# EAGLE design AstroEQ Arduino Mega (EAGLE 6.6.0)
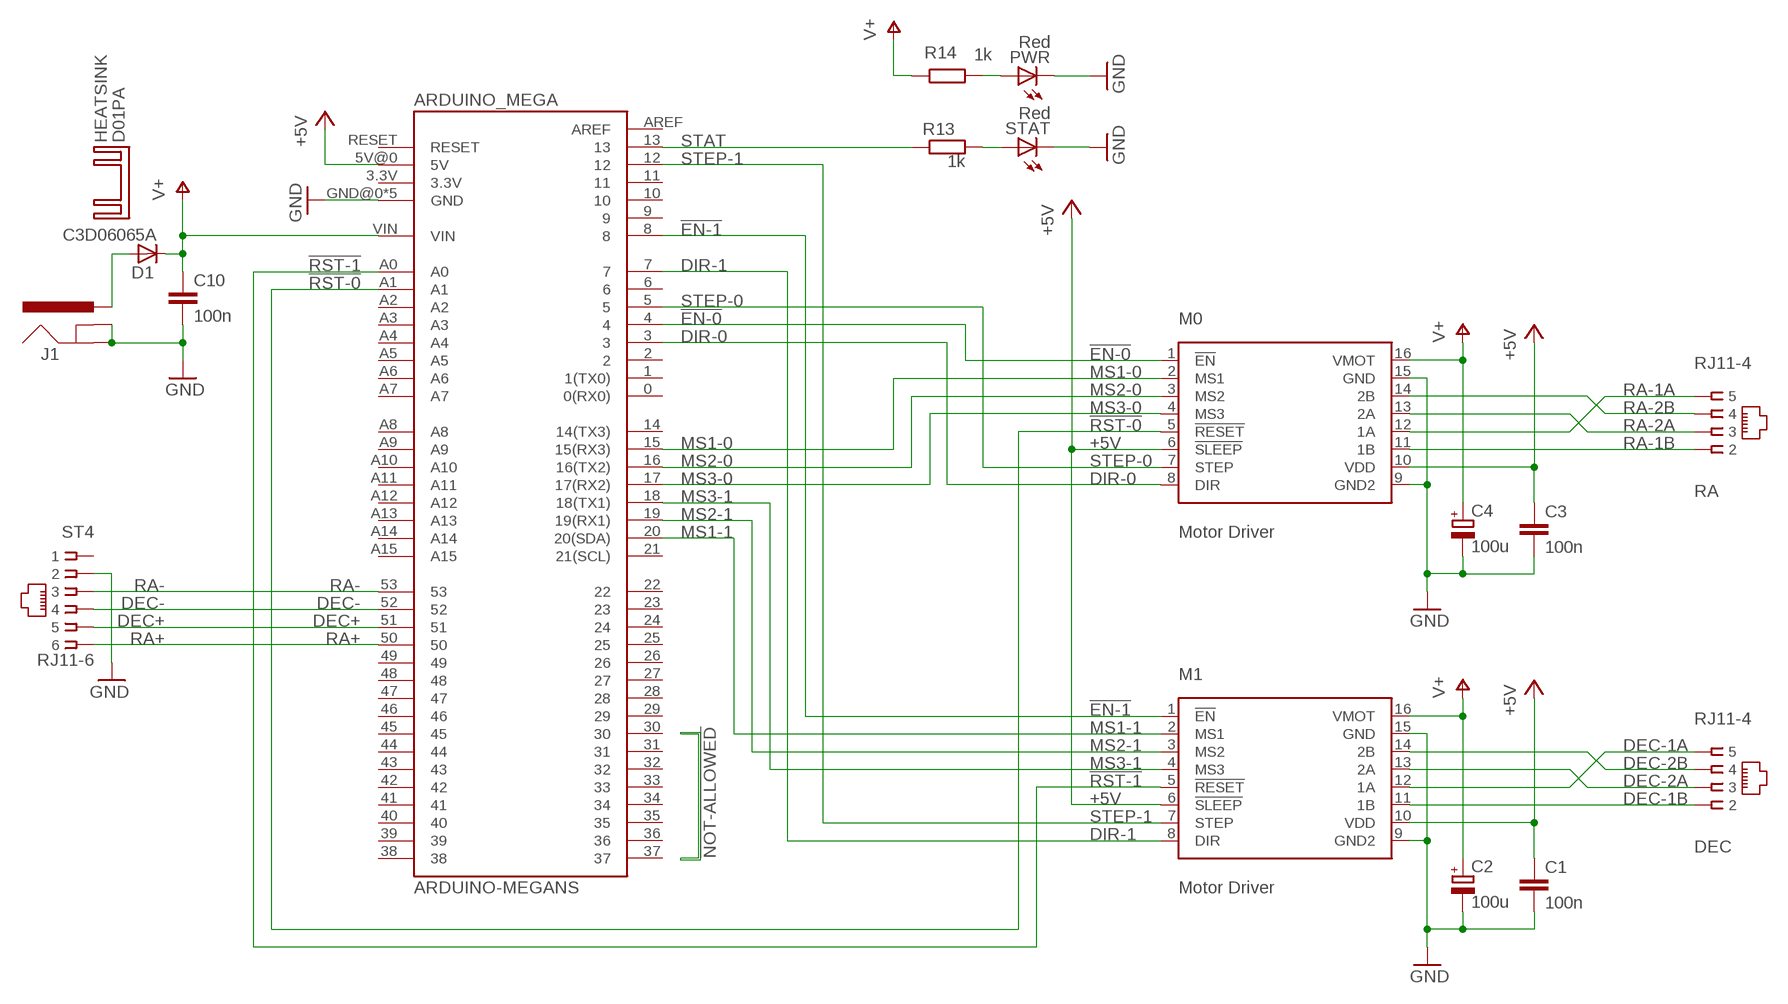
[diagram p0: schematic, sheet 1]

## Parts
ARDUINO_MEGA  ARDUINO-MEGANS  [ARDUINO_MEGA_NS]
C1  100n  C-EU025-024X044  [C025-024X044]
C2  100u  CPOL-EUE2.5-7  [E2,5-7]
C3  100n  C-EU025-024X044  [C025-024X044]
C4  100u  CPOL-EUE2.5-7  [E2,5-7]
C10  100n  C-EU025-024X044  [C025-024X044]
D1  C3D06065A  MUR820VERT  [TO220ACS]
DEC  RJ11-4  [RJ11-NO_SHIELD-4]
HEATSINK  D01PA  [D01PA]
J1  POWER_JACKPTH  [POWER_JACK_PTH]
M0  Motor Driver  A4983CARRIER  [DIP16-W]
M1  Motor Driver  A4983CARRIER  [DIP16-W]
PWR  Red  LED3MM  [LED3MM]
R13  1k  R-EU_0204/5  [0204/5]
R14  1k  R-EU_0204/7  [0204/7]
RA  RJ11-4  [RJ11-NO_SHIELD-4]
ST4  RJ11-6  RJ11-2L-B  [RJ11-NO_SHIELD]
STAT  Red  LED3MM  [LED3MM]

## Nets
!EN-0: ARDUINO_MEGA.4 M0.1(!EN)
!EN-1: ARDUINO_MEGA.8 M1.1(!EN)
!RST-0: ARDUINO_MEGA.A1 M0.5(!RESET)
!RST-1: ARDUINO_MEGA.A0 M1.5(!RESET)
+5V: ARDUINO_MEGA.5V@0(5V) C1.1 C3.1 M0.6(!SLEEP) M0.10(VDD) M1.6(!SLEEP) M1.10(VDD)
DEC+: ARDUINO_MEGA.51 ST4.5
DEC-: ARDUINO_MEGA.52 ST4.4
DEC-1A: DEC.5 M1.12(1A)
DEC-1B: DEC.2 M1.11(1B)
DEC-2A: DEC.3 M1.13(2A)
DEC-2B: DEC.4 M1.14(2B)
DIR-0: ARDUINO_MEGA.3 M0.8(DIR)
DIR-1: ARDUINO_MEGA.7 M1.8(DIR)
GND: ARDUINO_MEGA.GND@0(GND) ARDUINO_MEGA.GND@1(GND) ARDUINO_MEGA.GND@2(GND) ARDUINO_MEGA.GND@3(GND) ARDUINO_MEGA.GND@4(GND) C1.2 C2.- C3.2 C4.- C10.2 J1.GND J1.GNDBREAK M0.9(GND2) M0.15(GND) M1.9(GND2) M1.15(GND) PWR.K(C) ST4.2 STAT.K(C)
MS1-0: ARDUINO_MEGA.15(15(RX3)) M0.2(MS1)
MS1-1: ARDUINO_MEGA.20(20(SDA)) M1.2(MS1)
MS2-0: ARDUINO_MEGA.16(16(TX2)) M0.3(MS2)
MS2-1: ARDUINO_MEGA.19(19(RX1)) M1.3(MS2)
MS3-0: ARDUINO_MEGA.17(17(RX2)) M0.4(MS3)
MS3-1: ARDUINO_MEGA.18(18(TX1)) M1.4(MS3)
PWRLED: PWR.A R14.2
RA+: ARDUINO_MEGA.50 ST4.6
RA-: ARDUINO_MEGA.53 ST4.3
RA-1A: M0.12(1A) RA.5
RA-1B: M0.11(1B) RA.2
RA-2A: M0.13(2A) RA.3
RA-2B: M0.14(2B) RA.4
STAT: ARDUINO_MEGA.13 R13.1
STATLED: R13.2 STAT.A
STEP-0: ARDUINO_MEGA.5 M0.7(STEP)
STEP-1: ARDUINO_MEGA.12 M1.7(STEP)
V+: ARDUINO_MEGA.VIN C2.+ C4.+ C10.1 D1.C M0.16(VMOT) M1.16(VMOT) R14.1
VIN: D1.A J1.PWR
Unconnected: ARDUINO_MEGA.0(0(RX0)) ARDUINO_MEGA.1(1(TX0)) ARDUINO_MEGA.2 ARDUINO_MEGA.3.3V ARDUINO_MEGA.6 ARDUINO_MEGA.9 ARDUINO_MEGA.10 ARDUINO_MEGA.11 ARDUINO_MEGA.14(14(TX3)) ARDUINO_MEGA.21(21(SCL)) ARDUINO_MEGA.22 ARDUINO_MEGA.23 ARDUINO_MEGA.24 ARDUINO_MEGA.25 ARDUINO_MEGA.26 ARDUINO_MEGA.27 ARDUINO_MEGA.28 ARDUINO_MEGA.29 ARDUINO_MEGA.30 ARDUINO_MEGA.31 ARDUINO_MEGA.32 ARDUINO_MEGA.33 ARDUINO_MEGA.34 ARDUINO_MEGA.35 ARDUINO_MEGA.36 ARDUINO_MEGA.37 ARDUINO_MEGA.38 ARDUINO_MEGA.39 ARDUINO_MEGA.40 ARDUINO_MEGA.41 ARDUINO_MEGA.42 ARDUINO_MEGA.43 ARDUINO_MEGA.44 ARDUINO_MEGA.45 ARDUINO_MEGA.46 ARDUINO_MEGA.47 ARDUINO_MEGA.48 ARDUINO_MEGA.49 ARDUINO_MEGA.A2 ARDUINO_MEGA.A3 ARDUINO_MEGA.A4 ARDUINO_MEGA.A5 ARDUINO_MEGA.A6 ARDUINO_MEGA.A7 ARDUINO_MEGA.A8 ARDUINO_MEGA.A9 ARDUINO_MEGA.A10 ARDUINO_MEGA.A11 ARDUINO_MEGA.A12 ARDUINO_MEGA.A13 ARDUINO_MEGA.A14 ARDUINO_MEGA.A15 ARDUINO_MEGA.AREF ARDUINO_MEGA.RESET ST4.1

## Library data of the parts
ARDUINO_MEGA = SparkFun:ARDUINO-MEGA: Arduino Mega footprint connections
C1 C3 C10 = resistor:C-EU: CAPACITOR, European symbol; MF: AVX; MPN: SR205C104KAR; OC_FARNELL: 1100367
C2 C4 = resistor:CPOL-EU: POLARIZED CAPACITOR, European symbol; MF: MULTICOMP; MPN: MCGPR25V107M6.3X11; OC_FARNELL: 9451188
D1 = diode:MUR820: DIODE; MF: CREE; MPN: C3D06065A; OC_FARNELL: 1864928
DEC RA = con-tycoelectronics:RJ11-4; MF: MOLEX; MPN: 95501-2641; OC_FARNELL: 1560166
HEATSINK = heatsink:D01PA: HEATSINK
J1 = SparkFun:POWER_JACK: Power Jack This is the standard 5.5mm barrel jack for power. The PTH is the most common, proven, reliable, footprint. All others are experimental. The Slot footprint only works if the mill layer is transmitted to the PCB fab house so be warned. Spark Fun Electronics SKU : PRT-00119. Mating wall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; MF: MULTICOMP; MPN: MJ-179PH; OC_FARNELL: 1737246
M0 M1 = A4983Carrier:A4983CARRIER; MF: SAMTEC; MPN: CES-116-01-T-S; OC_FARNELL: 1667522
PWR STAT = led:LED: LED; MF: KINGBRIGHT; MPN: L-424HDT; OC_FARNELL: 1142499
R13 R14 = rcl:R-EU_: RESISTOR, European symbol; MF: MULTICOMP; MPN: MF12 1K; OC_FARNELL: 9342400
ST4 = con-tycoelectronics:RJ11: CORCOM Modular RJ Jacks No Shield Source: www.tycoelectronics.com .. ENG_DS_1654001_1099_RJ_L_0507.pdf; MF: TYCO ELECTRONICS; MPN: RJ11-2L-B; OC_FARNELL: unknown; OC_NEWARK: 83F4463

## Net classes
1 power: width 0.61 mm, drill 0.711 mm, clearance 0.203 mm
2 gnd: width 0.305 mm, drill 0.711 mm, clearance 0.203 mm
3 usbvcc: width 0.508 mm, drill 0.711 mm, clearance 0.203 mm

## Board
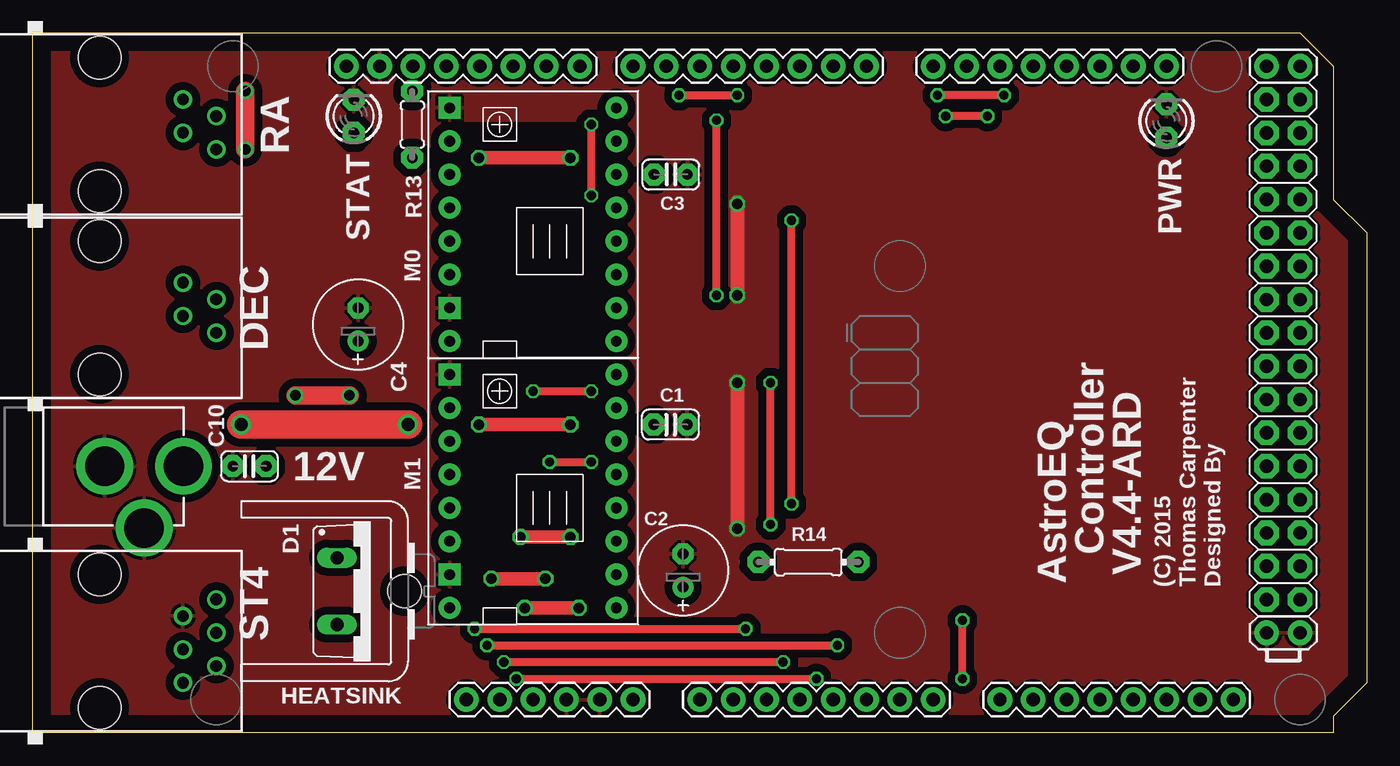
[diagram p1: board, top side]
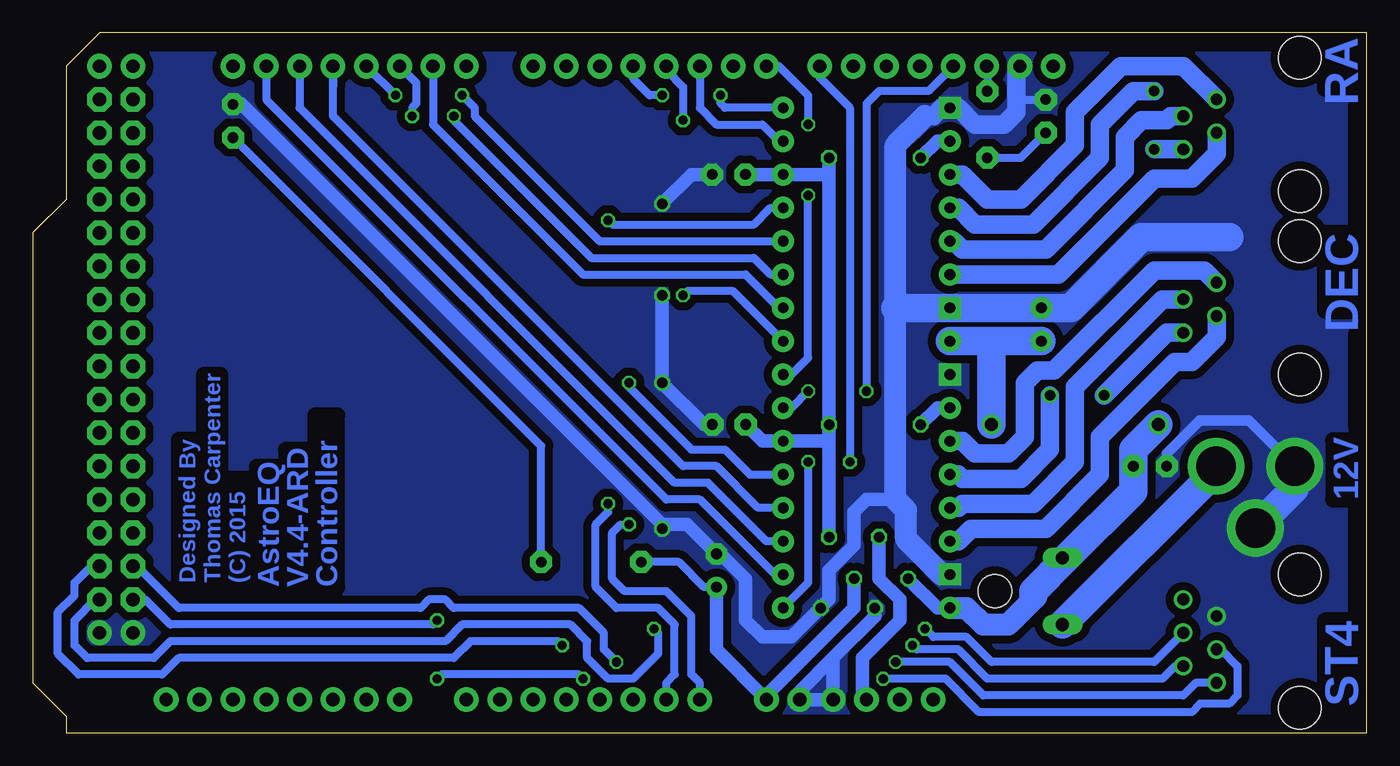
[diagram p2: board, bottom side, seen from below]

Size 101.6 x 53.34 mm. Coordinates in mm from the lower left corner, seen from the top.
Copper layers (1*16): Top 0.035mm / dielectric 1.5mm / Bottom 0.035mm
Design rules "default *": minimum track width 6mil, minimum drill 12mil, track to track 6mil, track to pad 6mil, pad to pad 6mil, via to via 6mil, smd to smd 0mil, copper to edge 12mil, drill to drill 10mil, minimum pad ring 10mil, minimum via ring 6mil, stop-mask expansion 2mil, vias tented up to drill 1mm, thermal gap 10mil
tRestrict: 8 lines
bRestrict: 10 lines

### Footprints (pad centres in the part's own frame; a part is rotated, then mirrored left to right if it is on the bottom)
ARDUINO_MEGA_NS = drill 1.016 pad 1.88: 0 63.5,50.8; 1 60.96,50.8; 2 58.42,50.8; 3 55.88,50.8; 3.3V 35.56,2.54; 4 53.34,50.8; 5 50.8,50.8; 5V@0 38.1,2.54; 5V@1 93.98,50.8; 5V@2 96.52,50.8; 6 48.26,50.8; 7 45.72,50.8; 8 41.656,50.8; 9 39.116,50.8; 10 36.576,50.8; 11 34.036,50.8; 12 31.496,50.8; 13 28.956,50.8; 14 68.58,50.8; 15 71.12,50.8; 16 73.66,50.8; 17 76.2,50.8; 18 78.74,50.8; 19 81.28,50.8; 20 83.82,50.8; 21 86.36,50.8; A0 50.8,2.54; A1 53.34,2.54; A2 55.88,2.54; A3 58.42,2.54; A4 60.96,2.54; A5 63.5,2.54; A6 66.04,2.54; A7 68.58,2.54; A8 73.66,2.54; A9 76.2,2.54; A10 78.74,2.54; A11 81.28,2.54; A12 83.82,2.54; A13 86.36,2.54; A14 88.9,2.54; A15 91.44,2.54; AREF 23.876,50.8; GND@0 40.64,2.54; GND@1 43.18,2.54; GND@2 93.98,7.62; GND@3 96.52,7.62; GND@4 26.416,50.8; RESET 33.02,2.54; VIN 45.72,2.54 | drill 1.016 pad 1.88 octagon: 22 93.98,48.26; 23 96.52,48.26; 24 93.98,45.72; 25 96.52,45.72; 26 93.98,43.18; 27 96.52,43.18; 28 93.98,40.64; 29 96.52,40.64; 30 93.98,38.1; 31 96.52,38.1; 32 93.98,35.56; 33 96.52,35.56; 34 93.98,33.02; 35 96.52,33.02; 36 93.98,30.48; 37 96.52,30.48; 38 93.98,27.94; 39 96.52,27.94; 40 93.98,25.4; 41 96.52,25.4; 42 93.98,22.86; 43 96.52,22.86; 44 93.98,20.32; 45 96.52,20.32; 46 93.98,17.78; 47 96.52,17.78; 48 93.98,15.24; 49 96.52,15.24; 50 93.98,12.7; 51 96.52,12.7; 52 93.98,10.16; 53 96.52,10.16
C025-024X044 = drill 0.813 pad 1.676 octagon: 1 -1.27,0; 2 1.27,0
E2,5-7 = drill 0.813 pad 1.6: + -1.27,0 | drill 0.813 pad 1.6 octagon: - 1.27,0
TO220ACS = drill 1.016 long: A 2.54,-2.54; C -2.54,-2.54
RJ11-NO_SHIELD-4 = drill 0.9 pad 1.4: 2 -1.905,6.35; 3 -0.635,8.89; 4 0.635,6.35; 5 1.905,8.89 | hole 3.251: -5.08,0; 5.08,0
D01PA = hole 2.54: 0,-1.016
POWER_JACK_PTH = drill 2.997 pad 4.318: GND 0,7.7; GNDBREAK 4.7,10.7; PWR 0,13.7
DIP16-W = drill 0.813 pad 1.676: 1 -8.89,-6.35; 2 -6.35,-6.35; 3 -3.81,-6.35; 4 -1.27,-6.35; 5 1.27,-6.35; 6 3.81,-6.35; 7 6.35,-6.35; 8 8.89,-6.35; 10 6.35,6.35; 11 3.81,6.35; 12 1.27,6.35; 13 -1.27,6.35; 14 -3.81,6.35; 16 -8.89,6.35 | drill 0.813 pad 1.676 square: 9 8.89,6.35; 15 -6.35,6.35
LED3MM = drill 0.813 pad 1.676 octagon: A -1.27,0; K 1.27,0
0204/5 = drill 0.813 pad 1.676 octagon: 1 -2.54,0; 2 2.54,0
0204/7 = drill 0.813 pad 1.676 octagon: 1 -3.81,0; 2 3.81,0
RJ11-NO_SHIELD = drill 0.9 pad 1.4: 1 -3.175,8.89; 2 -1.905,6.35; 3 -0.635,8.89; 4 0.635,6.35; 5 1.905,8.89; 6 3.175,6.35 | hole 3.251: -5.08,0; 5.08,0

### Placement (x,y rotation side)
ARDUINO_MEGA  0,0 0 top
C1  48.57,23.5 0 top
C2  49.53,12.37 90 top
C3  48.59,42.55 0 top
C4  24.77,31.11 90 top
C10  16.5,20.32 180 top
D1  25.72,10.79 270 top
DEC  5.08,32.4 270 top
HEATSINK  27.3,10.79 90 top
J1  -2.22,20.31 270 top
M0  38.1,38.73 90 top
M1  38.1,18.41 90 top
PWR  86.35,46.62 90 top
R13  28.9,46.35 270 top
R14  59.06,13.02 0 top
RA  5.08,46.37 270 top
ST4  5.08,7 270 top
STAT  24.45,46.99 90 top

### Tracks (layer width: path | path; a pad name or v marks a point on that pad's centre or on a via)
!EN-0  (via drill 0.7)
  Top 0.61: v52.07,33.34 v52.07,46.67
  Bottom 0.61: ARDUINO_MEGA.4 53.34,50.48 52.07,49.21 v52.07,46.67 | M0.1 48.26,33.66 51.75,33.66 v52.07,33.34
!EN-1  (via drill 0.7)
  Top 0.61: v39.37,20.64 v42.55,20.64
  Bottom 0.61: ARDUINO_MEGA.8 41.66,49.91 39.37,47.62 v39.37,20.64 | v42.55,20.64 42.55,11.43 M1.1
!RST-0  (via drill 0.7)
  Top 0.61: v57.78,17.46 v57.78,39.05
  Bottom 0.61: ARDUINO_MEGA.A1 53.34,3.81 52.7,4.45 52.7,8.26 53.98,9.53 57.15,9.53 58.74,11.11 58.74,15.88 57.78,16.83 v57.78,17.46 | v57.78,39.05 57.47,38.73 46.67,38.73 45.4,40.01 M0.5
!RST-1  (via drill 0.7)
  Top 0.61: v56.2,15.88 v56.2,26.67
  Bottom 0.61: ARDUINO_MEGA.A0 50.8,3.81 51.44,4.45 51.44,8.89 53.34,10.79 56.52,10.79 57.47,11.75 57.47,15.24 56.83,15.88 v56.2,15.88 | v56.2,26.67 56.2,26.35 51.44,21.59 48.9,21.59 46.99,19.68 M1.5
+5V  (via drill 0.8)
  Top 1.016: v33.97,23.5 v40.96,23.5 | v33.97,43.81 v40.96,43.81 | v37.15,14.92 v40.96,14.92
  Bottom 1.016: M1.10 32.7,24.77 v33.97,23.5 | 40.96,22.23 v40.96,23.5 40.96,42.55 | M0.10 32.7,45.09 v33.97,43.81 | v40.96,43.81 40.96,42.55 | 40.96,42.55 M0.6 C3.1 | 40.96,22.23 M1.6 46.03,22.23 C1.1 | v37.15,14.92 37.15,11.75 35.56,10.16 35.56,8.57 38.42,5.71 38.42,2.86 ARDUINO_MEGA.5V@0 | v40.96,14.92 40.96,22.23
DEC+  (via drill 0.7)
  Top 0.61: v34.61,6.67 v61.28,6.67
  Bottom 0.61: ST4.5 14.61,5.08 15.56,4.13 28.89,4.13 31.11,6.35 34.29,6.35 v34.61,6.67 | v61.28,6.67 61.59,6.99 68.26,6.99 69.53,5.71 90.49,5.71 91.76,4.45 98.11,4.45 99.69,6.03 99.69,9.21 98.42,10.48 98.42,11.43 97.16,12.7 ARDUINO_MEGA.51
DEC-  (via drill 0.7)
  Top 0.61: v36.83,4.13 v59.69,4.13 | v70.8,4.13 v70.8,8.57
  Bottom 0.61: ST4.4 11.11,6.35 9.84,5.08 9.84,2.86 10.48,2.22 12.7,2.22 13.34,1.59 29.53,1.59 32.07,4.13 v36.83,4.13 | v59.69,4.13 60.01,4.45 70.48,4.45 v70.8,4.13 | v70.8,8.57 71.12,8.26 91.12,8.26 93.03,10.16 ARDUINO_MEGA.52
DEC-1A  (via drill 0.8)
  Top 1.422: v24.13,25.72 v20,25.72
  Bottom 1.422: v24.13,25.72 24.13,21.59 26.35,19.37 30.8,19.37 31.11,19.68 M1.12 | v20,25.72 15.23,30.49 DEC.5
DEC-1B
  Bottom 1.422: DEC.2 12.38,35.24 16.19,35.24 23.81,27.62 25.08,27.62 26.04,26.67 26.04,22.54 27.3,21.27 29.84,21.27 30.8,22.23 M1.11
DEC-2A
  Bottom 1.422: M1.13 31.11,17.14 30.8,17.46 25.4,17.46 22.23,20.64 22.23,26.35 15.55,33.03 DEC.3
DEC-2B
  Bottom 1.422: DEC.4 11.43,30.16 13.34,28.26 14.61,28.26 20.32,22.54 20.32,19.68 24.45,15.56 30.16,15.56 31.11,14.61 M1.14
DIR-0  (via drill 0.7)
  Top 0.61: v49.21,48.58 v53.66,48.58
  Bottom 0.61: M0.8 48.9,47.62 49.21,47.94 v49.21,48.58 | v53.66,48.58 54.61,48.58 55.88,49.85 ARDUINO_MEGA.3
DIR-1  (via drill 0.7)
  Top 0.61: v42.55,40.96 v42.55,46.35
  Bottom 0.61: ARDUINO_MEGA.7 44.77,50.8 42.55,48.58 v42.55,46.35 | M1.8 43.81,27.3 42.55,28.57 v42.55,40.96
GND  (via drill 0.8)
  Top 1.016: v37.47,9.53 v41.59,9.53 | v53.66,15.56 v53.66,26.67 | v53.66,33.34 v53.66,40.32
  Bottom 0.61: ST4.2 11.75,8.89 | 26.67,48.26 STAT.K
  Bottom 0.813: C10.2 15.23,21.28 12.7,23.81 8.98,23.81 J1.GND
  Bottom 1.016: 40.64,5.71 ARDUINO_MEGA.GND@0 ARDUINO_MEGA.GND@1 43.18,3.17 40.64,5.71 | 40.64,5.71 37.47,8.89 v37.47,9.53 | 35.88,17.78 38.1,17.78 39.05,16.83 39.05,14.29 40.96,12.38 40.96,10.16 v41.59,9.53 43.81,7.3 46.04,7.3 47.31,8.57 47.31,11.75 49.2,13.64 C2.- 51.76,15.88 53.66,15.88 | 53.66,15.88 85.72,47.94 86.36,47.94 | v53.66,40.32 51.44,42.55 C3.2 | v53.66,15.56 53.66,15.88 | v53.66,33.34 v53.66,26.67 50.48,23.5 C1.2
  Bottom 1.422: 33.66,46.99 33.02,46.99 32.38,47.62 M0.9 31.11,47.62 29.84,46.35 27.62,46.35 26.67,47.31 26.67,48.26 26.67,50.55 ARDUINO_MEGA.GND@4
  Bottom 1.676: M1.15 32.38,12.06 35.08,14.76 35.08,16.99 35.88,17.78 35.88,32.38 35.88,44.77 33.66,46.99
  Bottom 2.184: J1.GND 5.48,18.61 J1.GNDBREAK | 10.48,37.78 17.14,37.78 22.54,32.38 M0.15 35.88,32.38
  pour Bottom (isolate 0.61, no thermals): -0.64,-0.64 102.87,-0.64 102.87,53.98 -0.64,53.98
  pour Top (isolate 0.61): -0.64,-0.64 102.87,-0.64 102.87,53.98 31.75,53.98 31.75,46.67 44.13,46.67 44.13,8.26 31.75,8.26 31.75,53.98 -0.64,53.98
MS1-0
  Bottom 0.61: ARDUINO_MEGA.15 71.12,46.35 59.69,34.92 47.31,34.92 44.77,32.38 M0.2
MS1-1
  Bottom 0.61: M1.2 45.09,12.06 50.8,17.78 53.34,17.78 83.82,48.26 ARDUINO_MEGA.20
MS2-0  (via drill 0.7)
  Top 0.61: v72.71,46.99 v69.53,46.99
  Bottom 0.61: ARDUINO_MEGA.16 72.39,49.53 72.39,47.94 72.71,47.62 v72.71,46.99 | v69.53,46.99 69.53,46.67 59.05,36.2 46.67,36.2 45.4,34.92 M0.3
MS2-1
  Bottom 0.61: M1.3 45.72,14.61 50.16,19.05 52.7,19.05 81.28,47.62 ARDUINO_MEGA.19
MS3-0  (via drill 0.7)
  Top 0.61: v73.98,48.58 v68.9,48.58
  Bottom 0.61: ARDUINO_MEGA.17 v73.98,48.58 | v68.9,48.58 67.94,47.62 67.94,46.99 58.42,37.47 M0.4
MS3-1
  Bottom 0.61: M1.4 46.35,17.14 49.53,20.32 52.07,20.32 78.74,46.99 ARDUINO_MEGA.18 78.74,49.21
PWRLED
  Bottom 0.61: R14.2 62.88,21.88 PWR.A
RA+  (via drill 0.7)
  Top 0.61: v35.88,5.4 v57.15,5.4
  Bottom 0.61: ST4.6 13.02,3.81 13.97,2.86 29.21,2.86 31.75,5.4 v35.88,5.4 | v57.15,5.4 58.1,6.35 58.1,7.62 60.01,9.53 69.53,9.53 70.17,10.16 71.44,10.16 72.07,9.53 90.49,9.53 93.66,12.7 ARDUINO_MEGA.50
RA-  (via drill 0.7)
  Top 0.61: v33.66,7.94 v54.29,7.94
  Bottom 0.61: ST4.3 16.19,5.4 28.57,5.4 30.48,7.3 33.02,7.3 v33.66,7.94 | v54.29,7.94 53.98,7.62 53.98,6.03 55.88,4.13 57.78,4.13 59.37,5.71 59.37,6.99 60.64,8.26 68.9,8.26 70.17,6.99 91.12,6.99 92.39,5.71 97.47,5.71 98.42,6.67 98.42,8.57 96.84,10.16 ARDUINO_MEGA.53
RA-1A  (via drill 0.8)
  Top 1.422: v16.19,48.9 v16.19,44.46
  Bottom 1.422: v16.19,44.46 RA.5 | v16.19,48.9 17.78,48.9 20.32,46.35 20.32,43.81 25.4,38.73 29.84,38.73 31.11,40.01 M0.12
RA-1B
  Bottom 1.422: RA.2 13.96,50.8 18.73,50.8 22.23,47.31 22.23,44.77 26.35,40.64 28.89,40.64 30.8,42.55 M0.11
RA-2A
  Bottom 1.422: RA.3 14.92,46.99 15.24,46.67 17.14,46.67 18.41,45.4 18.41,42.86 24.45,36.83 30.8,36.83 31.43,37.47 M0.13
RA-2B  (1 unrouted)
  Bottom 1.422: RA.4 11.43,44.13 13.34,42.23 16.19,42.23 23.5,34.92 M0.14
STAT
  Bottom 0.61: ARDUINO_MEGA.13 28.9,50.75 R13.1
STATLED
  Bottom 0.61: R13.2 26.35,43.81 STAT.A
STEP-0
  Bottom 0.61: ARDUINO_MEGA.5 50.8,47.62 49.53,46.35 46.04,46.35 44.77,45.09 M0.7
STEP-1  (via drill 0.7)
  Top 0.61: v38.1,26.04 v42.55,26.04
  Bottom 0.61: v38.1,26.04 38.1,47.94 37.15,48.9 33.4,48.9 ARDUINO_MEGA.12 | v42.55,26.04 43.81,24.77 M1.7
V+  (via drill 0.8, 1)
  Top 1.016: v34.92,11.75 v39.05,11.75
  Top 2.184: v15.88,23.5 v28.57,23.5
  Bottom 0.61: C2.+ 50.47,11.1 52.39,13.02 R14.1
  Bottom 0.813: C10.1
  Bottom 1.016: v39.05,11.75 39.05,9.53 45.72,2.86 ARDUINO_MEGA.VIN 49.53,6.35 C2.+ | M1.16 32.7,9.53 v34.92,11.75
  Bottom 1.676: M1.16 30.48,9.53 29.21,8.26 27.3,8.26 25.4,10.16 25.4,10.48 | 22.86,13.34 D1.C
  Bottom 2.184: v15.88,23.5 17.78,21.59 C10.1 17.78,18.41 22.86,13.34 25.4,10.79 25.4,10.48 | v28.57,23.5 28.57,29.84 | 28.57,29.84 M0.16 | 28.57,29.84 C4.+
VIN
  Bottom 2.184: 11.16,20.27 11.27,20.16 | 11.27,20.16 D1.A | J1.PWR 11.42,20.31 11.27,20.16

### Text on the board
Bottom: RA | DEC | 12V | Controller | V4.4-ARD | AstroEQ | (C) 2015 | Thomas Carpenter | Designed By | ST4
tNames: Controller | V4.4-ARD | AstroEQ | 12V | (C) 2015 | Thomas Carpenter | Designed By
tValues: Thick Wire! | 4988 | Markings under motor drivers / show location of Potentiometers / on the Pololu Boards depending / on which chip they use. | Sq Pad | 8824/5 | 4988 | Thick Wire! | Sq Pad | 8824/5
Reference: This board design is for Arduino Mega based AstroEQ controllers. | It is a 2 Layer board designed to be sent for manufacture. The AstroEQ-ARD-Gerber.zip file contains the required gerber files. | I use iteadstudio.com 10cm x 10cm prototype service, selecting 1.6mm thick, HASL, 100% electrical check | It can also be home etched as a 1 Layer board, using only the bottom, and making sure all white lines are connected with wires. | For printing the silkscreen to paper, you should only have TNames, TValues and Dimension layers visible.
